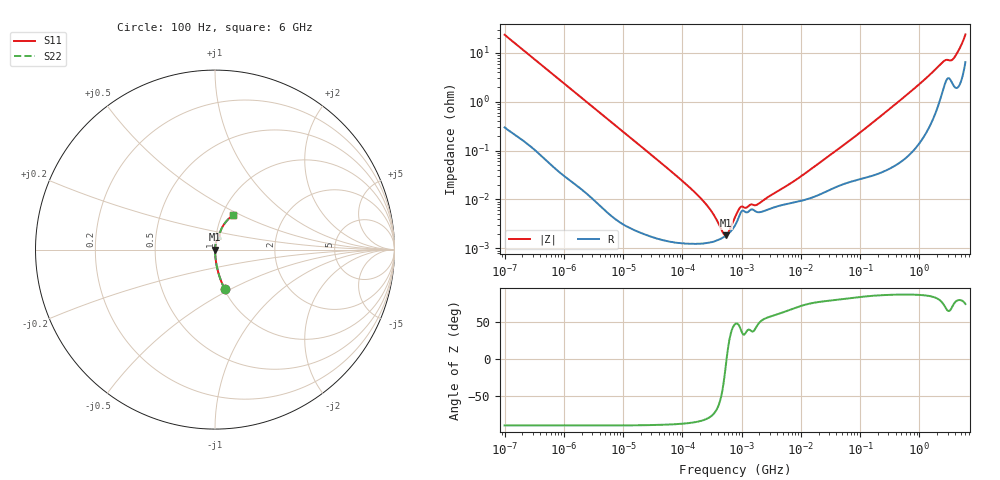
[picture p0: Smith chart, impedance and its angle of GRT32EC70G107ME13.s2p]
!Murata Part Number: GRT32EC70G107ME13
!These Parameters are Measured in Series Mode Connection
!Data Generated on Jun 19, 2026
!  o--ll--o
!Port1  Port2
!  o------o
!Operation Temp=25[degC], DC Bias Voltage=0[V]
!Freq. Start=100[Hz] Stop=6[GHz] 401[Steps]
# Hz S RI R 50
!Freq.(Hz) S11(Real) S11(Imag) S21(Real) S21(Imag) S12(Real) S12(Imag) S22(Real) S22(Imag)
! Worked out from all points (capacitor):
!   401 points, 100 Hz to 6 GHz, reference 50 ohm
!   read as one part in series: C = 67.4 uF near 109 Hz
!   lowest |Z| = 1.83 mohm at 541.4 kHz (marker M1)
!   series resonance near 558.3 kHz, so ESL is about 1.2 nH
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100  0.0551 -0.2219  0.9449 0.2219  0.9449 0.2219  0.0551 -0.2219
187  0.0174 -0.1241  0.9826 0.1241  0.9826 0.1241  0.0174 -0.1241
350  0.00554 -0.0676  0.9945 0.0676  0.9945 0.0676  0.00554 -0.0676
2008  0.000304 -0.012  0.9997 0.012  0.9997 0.012  0.000304 -0.012
40335  1.58e-05 -0.000607  1 0.000607  1 0.000607  1.58e-05 -0.000607
103284  1.27e-05 -0.000231  1 0.000231  1 0.000231  1.27e-05 -0.000231
211427  1.25e-05 -0.000101  1 0.000101  1 0.000101  1.25e-05 -0.000101
241822  1.27e-05 -8.36e-05  1 8.36e-05  1 8.36e-05  1.27e-05 -8.36e-05
541393  1.81e-05 -2.8e-06  1 2.8e-06  1 2.8e-06  1.81e-05 -2.8e-06
774597  2.93e-05 3.16e-05  1 -3.16e-05  1 -3.16e-05  2.93e-05 3.16e-05
2481164  5.88e-05 8.28e-05  0.9999 -8.28e-05  0.9999 -8.28e-05  5.88e-05 8.28e-05
6948629  8.47e-05 0.000202  0.9999 -0.000202  0.9999 -0.000202  8.47e-05 0.000202
1.555665e7  0.00011 0.000422  0.9999 -0.000422  0.9999 -0.000422  0.00011 0.000422
8.154455e7  0.000247 0.00192  0.9998 -0.00192  0.9998 -0.00192  0.000247 0.00192
3.124326e8  0.000473 0.00706  0.9995 -0.00706  0.9995 -0.00706  0.000473 0.00706
1.094528e9  0.00226 0.0251  0.9977 -0.0251  0.9977 -0.0251  0.00226 0.0251
2.450438e9  0.0191 0.06  0.9809 -0.06  0.9809 -0.06  0.0191 0.06
2.802721e9  0.0294 0.0632  0.9706 -0.0632  0.9706 -0.0632  0.0294 0.0632
3.352442e9  0.0312 0.0604  0.9688 -0.0604  0.9688 -0.0604  0.0312 0.0604
3.666503e9  0.0271 0.0667  0.9729 -0.0667  0.9729 -0.0667  0.0271 0.0667
4.385646e9  0.0282 0.0946  0.9718 -0.0946  0.9718 -0.0946  0.0282 0.0946
6e9  0.1027 0.1938  0.8973 -0.1938  0.8973 -0.1938  0.1027 0.1938
